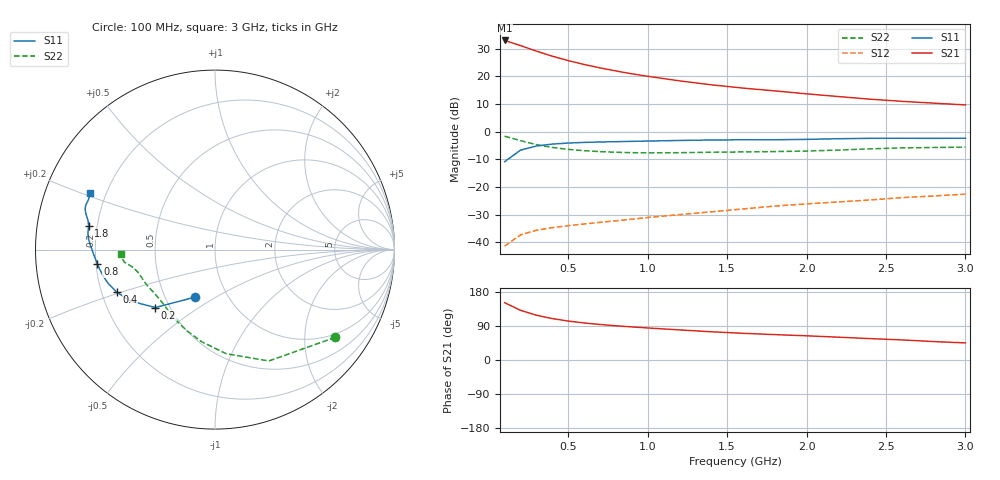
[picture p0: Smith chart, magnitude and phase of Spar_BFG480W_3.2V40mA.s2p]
! Filename: 3_240BFG480.001
! Title: BFG480W
! Bias: Vce=3.2V; Ic=40mA
! Company: NXP Semiconductors NL
! User: Quality&Reliability T&D
! Measure time: 10 Nov 1999 / 11:56:47
#  MHz  S  MA  R 50
! Freq  S11  S21  S12  S22  :
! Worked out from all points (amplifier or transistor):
!   20 points, 100 MHz to 3 GHz, reference 50 ohm
!   highest |S21| = 33.0 dB at 100 MHz (marker M1)
!   |S21| within 3 dB of that: start of sweep to 257.3 MHz
!   unconditionally stable (mu >= 1): 1.051 GHz to end of sweep
!   at 400 MHz: K = 0.58, MSG = 31.0 dB, |S12| = -34.7 dB
!   at 1.2 GHz: K = 1.04, MAG = 23.0 dB, |S12| = -30.0 dB
!   at 3 GHz: K = 1.07, MAG = 14.5 dB, |S12| = -22.6 dB
!   S11 on the Smith chart (normalised r, x): 100 MHz: 0.71, -0.41; 200 MHz: 0.42, -0.34; 400 MHz: 0.26, -0.19; 800 MHz: 0.21, -0.06; 1.8 GHz: 0.17, +0.09; 3 GHz: 0.14, +0.21
100  0.2862 -112.5  44.71 151.3  0.008498 67.3  0.8297 -36.1
200  0.4638 -135.9  36.12 131.1  0.01361 55.9  0.6893 -64.2
300  0.551 -148.7  28.69 118.2  0.01651 51.1  0.5836 -83.8
400  0.5965 -156.6  23.21 109.3  0.0184 49.8  0.5189 -98.2
500  0.6236 -162.3  19.35 102.8  0.01995 50.2  0.4792 -108.9
600  0.64 -166.6  16.45 97.8  0.02142 51.4  0.4538 -117.2
700  0.6512 -170.1  14.28 93.7  0.02293 53.3  0.4364 -123.7
800  0.66 -173.0  12.56 90.3  0.02446 55.2  0.4248 -129.2
900  0.6686 -175.6  11.17 87.3  0.02613 57.6  0.4176 -133.9
1000  0.6774 -178.0  10.05 84.6  0.02802 59.3  0.4144 -138.2
1200  0.6944 178.1  8.316 79.4  0.03161 62.3  0.4171 -145.3
1400  0.7074 175.1  7.053 74.5  0.0355 64.7  0.4251 -150.6
1600  0.7142 172.4  6.152 70.5  0.04002 66.9  0.4308 -154.6
1800  0.7157 169.5  5.471 67.0  0.04517 68.6  0.437 -158.7
2000  0.7263 167.0  4.842 63.9  0.04943 70.2  0.4465 -163.4
2200  0.7462 164.5  4.321 60.2  0.05366 70.9  0.4655 -167.5
2400  0.7589 162.6  3.875 56.4  0.05831 71.0  0.4897 -170.3
2600  0.761 160.8  3.542 53.1  0.06419 71.0  0.5087 -172.0
2800  0.7578 158.4  3.286 48.6  0.06878 70.1  0.5179 -174.1
3000  0.7629 155.7  3.051 45.1  0.07407 69.8  0.5255 -177.2
